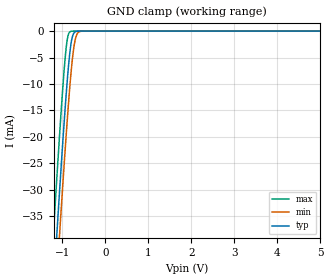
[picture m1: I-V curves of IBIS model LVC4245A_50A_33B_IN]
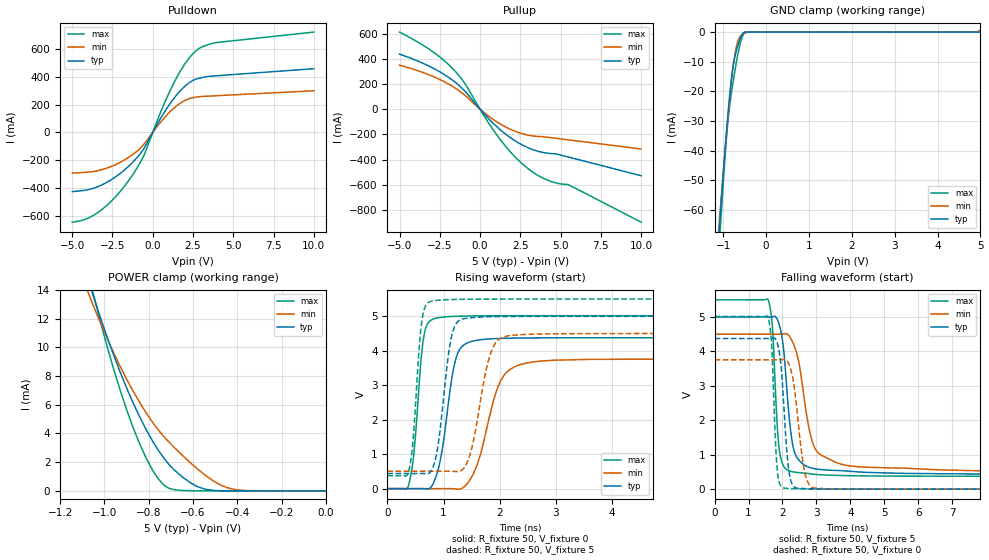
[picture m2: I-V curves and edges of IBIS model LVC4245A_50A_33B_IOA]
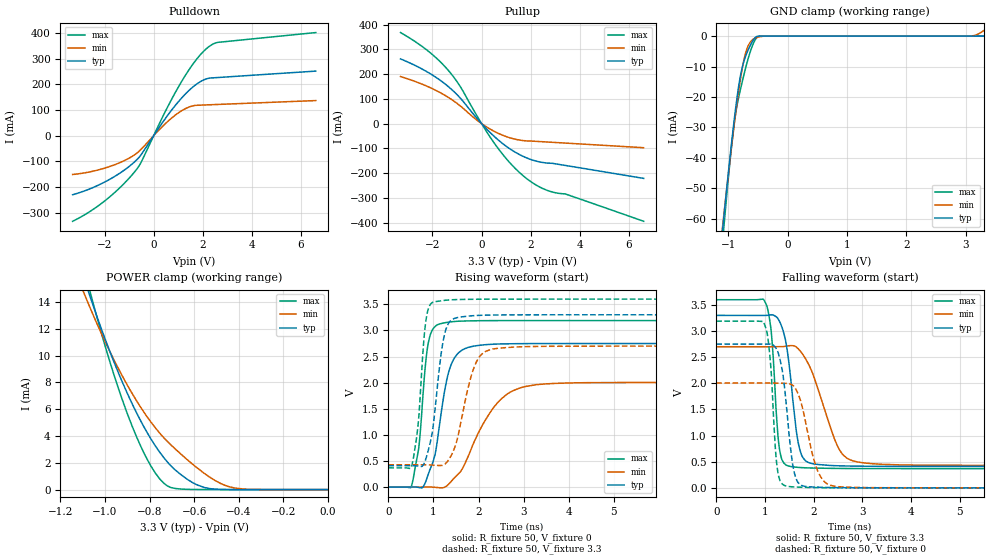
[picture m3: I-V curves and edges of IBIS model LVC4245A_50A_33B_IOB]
| TEXAS INSTRUMENTS INCORPORATED
| Standard Linear and Logic Group
| IBIS Model of SN74LVC4245A
| Octal Bus Transceiver And 3.3-V to 5-V Shifter With 3 state Outputs
| This file contains package information for the following:
|  SSOP 24-pin (DB) package as [Component] LVC4245A_DB
|  SOIC 24-pin (DW) package as [Component] LVC4245A_DW
|  TSSOP 24-pin (PW) package as [Component] LVC4245A_PW
| This device can be powered at the A side at the following Vcca:
|  5 volt Vcca
| This device can be powered at the B side at the following Vccb:
|  3.3 volt Vccb
| This file provides unique models under the [Model Selector] for each Vcc.
| For operation at a specific Vcc, select the appropriate model after each
| [Model Selector] keyword.
[IBIS Ver]   3.2
[Comment char]  |_char
[File Name]   sn74lvc4245a.ibs
[File Rev]   1.0 | b_die
[Date]   March 09, 2001
[Source]   Data created from TI-SPICE simulations at TI-SLL.
[Notes]   The following is an IBIS list for the LVC4245A.
   Please contact sllibis@ti.com with questions and
   comments concerning SLL IBIS models.
   - This device is a 3.3V to 5.0V level shifter, so
   we used the Model selector key word to distinguish
   each model with VCCA and VCCB.
[Disclaimer] Property of Texas Instruments Incorporated.  Unauthorized
   reproduction and/or distribution is strictly prohibited.
   This product is protected under copyright law.
   Created  2001, (C) Copyright  2001, Texas Instruments
   Incorporated, All Rights Reserved
   UNLESS THERE IS A SIGNED, WRITTEN AGREEMENT TO THE
   CONTRARY, TEXAS INSTRUMENTS (TI) IS PROVIDING THE IBIS
   MODELS  AND WITHOUT ANY WARRANTY, EXPRESSED OR
   IMPLIED.  TI assumes no liability for:
   1) the accuracy of the IBIS models provided to your
   company;
   2) the proper functioning of these IBIS Models in your
   design or for any resulting applications; or
   3) infringement of patents, copyrights or intellectual
   property rights resulting from your use of these IBIS
   models.
   TI provides IBIS Models as a service to our customers.
   You and your company shall not distribute, sell or give
   these models to anyone else without prior written
   permission from TI.
   TI reserves the right to make changes to our products or
   to discontinue any semiconductor product or service
   without notice, and advises our customers to obtain the
   latest version of relevant information to verify, before
   placing orders, that the information being relied on is
   current.
   Please be aware that your receipt and use of the IBIS
   information provided shall serve as acceptance of these
   terms and conditions.  If you do not accept these terms,
   you should return or destroy the IBIS models and any
   other accompanying information immediately.
| Component LVC4245A_DB 24-pin SSOP
[Component]   LVC4245A_DB
[Manufacturer]   Texas Instruments, Inc.
[Package]
|   typ   min   max
R_pkg   4.500e-02   4.000e-02   4.900e-02
L_pkg   3.668e-09   3.226e-09   4.415e-09
C_pkg   4.160e-13   3.490e-13   5.070e-13
[Pin]   signal_name   model_name   R_pin   L_pin   C_pin
1   VCCA   POWER   4.200e-02   4.299e-09   5.030e-13
2   DIR   LVC4245A_IN   4.000e-02   3.960e-09   4.990e-13
3   A1   LVC4245A_IOA   4.200e-02   3.775e-09   4.170e-13
4   A2   LVC4245A_IOA   4.700e-02   3.487e-09   3.690e-13
5   A3   LVC4245A_IOA   4.600e-02   3.347e-09   3.520e-13
6   A4   LVC4245A_IOA   4.900e-02   3.352e-09   3.710e-13
7   A5   LVC4245A_IOA   4.600e-02   3.226e-09   3.630e-13
8   A6   LVC4245A_IOA   4.700e-02   3.289e-09   3.490e-13
9   A7   LVC4245A_IOA   4.700e-02   3.347e-09   3.610e-13
10   A8   LVC4245A_IOA   4.100e-02   3.576e-09   4.090e-13
11   GND   GND   4.100e-02   3.995e-09   5.030e-13
12   GND   GND   4.500e-02   4.415e-09   5.070e-13
13   GND   GND   4.300e-02   4.337e-09   5.060e-13
14   B8   LVC4245A_IOB   4.200e-02   4.003e-09   5.040e-13
15   B7   LVC4245A_IOB   4.100e-02   3.686e-09   4.100e-13
16   B6   LVC4245A_IOB   4.800e-02   3.355e-09   3.490e-13
17   B5   LVC4245A_IOB   4.700e-02   3.301e-09   3.530e-13
18   B4   LVC4245A_IOB   4.800e-02   3.268e-09   3.660e-13
19   B3   LVC4245A_IOB   4.800e-02   3.269e-09   3.660e-13
20   B2   LVC4245A_IOB   4.700e-02   3.314e-09   3.490e-13
21   B1   LVC4245A_IOB   4.800e-02   3.399e-09   3.550e-13
22   OE   LVC4245A_IN   4.100e-02   3.688e-09   4.120e-13
23   VCCB   POWER   4.200e-02   4.003e-09   5.040e-13
24   VCCB   POWER   4.300e-02   4.347e-09   5.050e-13
| Component LVC4245A_DW 24-pin SOIC
[Component]   LVC4245A_DW
[Manufacturer]   Texas Instruments, Inc.
[Package]
|   typ   min   max
R_pkg   3.700e-02   3.000e-02   4.700e-02
L_pkg   5.146e-09   3.993e-09   6.885e-09
C_pkg   7.580e-13   5.120e-13   1.067e-12
[Pin]   signal_name   model_name   R_pin   L_pin   C_pin
1   VCCA   POWER   3.900e-02   6.885e-09   1.067e-12
2   DIR   LVC4245A_IN   4.200e-02   5.950e-09   9.580e-13
3   A1   LVC4245A_IOA   4.700e-02   5.317e-09   7.910e-13
4   A2   LVC4245A_IOA   3.100e-02   4.651e-09   6.110e-13
5   A3   LVC4245A_IOA   3.000e-02   3.993e-09   5.120e-13
6   A4   LVC4245A_IOA   3.000e-02   4.083e-09   6.110e-13
7   A5   LVC4245A_IOA   3.000e-02   4.083e-09   6.110e-13
8   A6   LVC4245A_IOA   3.000e-02   3.993e-09   5.120e-13
9   A7   LVC4245A_IOA   3.100e-02   4.652e-09   6.110e-13
10   A8   LVC4245A_IOA   4.700e-02   5.317e-09   7.910e-13
11   GND   GND   4.200e-02   5.950e-09   9.590e-13
12   GND   GND   3.900e-02   6.885e-09   1.067e-12
13   GND   GND   3.900e-02   6.885e-09   1.067e-12
14   B8   LVC4245A_IOB   4.200e-02   5.950e-09   9.590e-13
15   B7   LVC4245A_IOB   4.700e-02   5.317e-09   7.910e-13
16   B6   LVC4245A_IOB   3.100e-02   4.652e-09   6.110e-13
17   B5   LVC4245A_IOB   3.000e-02   3.993e-09   5.120e-13
18   B4   LVC4245A_IOB   3.000e-02   4.083e-09   6.100e-13
19   B3   LVC4245A_IOB   3.000e-02   4.083e-09   6.100e-13
20   B2   LVC4245A_IOB   3.000e-02   3.993e-09   5.120e-13
21   B1   LVC4245A_IOB   3.100e-02   4.651e-09   6.110e-13
22   OE   LVC4245A_IN   4.700e-02   5.317e-09   7.910e-13
23   VCCB   POWER   4.200e-02   5.950e-09   9.580e-13
24   VCCB   POWER   3.900e-02   6.885e-09   1.067e-12
| Component LVC4245A_PW 24-pin TSSOP
[Component]   LVC4245A_PW
[Manufacturer]   Texas Instruments, Inc.
[Package]
|   typ   min   max
R_pkg   3.900e-02   3.000e-02   4.600e-02
L_pkg   2.685e-09   2.367e-09   3.177e-09
C_pkg   3.200e-13   2.520e-13   4.340e-13
[Pin]   signal_name   model_name   R_pin   L_pin   C_pin
1   VCCA   POWER   3.700e-02   3.153e-09   4.340e-13
2   DIR   LVC4245A_IN   3.400e-02   2.629e-09   3.410e-13
3   A1   LVC4245A_IOA   3.200e-02   2.860e-09   3.470e-13
4   A2   LVC4245A_IOA   4.200e-02   2.741e-09   2.900e-13
5   A3   LVC4245A_IOA   4.600e-02   2.600e-09   2.620e-13
6   A4   LVC4245A_IOA   4.300e-02   2.414e-09   2.660e-13
7   A5   LVC4245A_IOA   4.200e-02   2.367e-09   2.620e-13
8   A6   LVC4245A_IOA   4.400e-02   2.461e-09   2.520e-13
9   A7   LVC4245A_IOA   4.200e-02   2.543e-09   2.740e-13
10   A8   LVC4245A_IOA   3.000e-02   2.616e-09   3.320e-13
11   GND   GND   3.700e-02   2.670e-09   3.460e-13
12   GND   GND   3.900e-02   3.177e-09   4.330e-13
13   GND   GND   3.700e-02   3.111e-09   4.310e-13
14   B8   LVC4245A_IOB   3.700e-02   2.656e-09   3.450e-13
15   B7   LVC4245A_IOB   3.100e-02   2.739e-09   3.400e-13
16   B6   LVC4245A_IOB   4.200e-02   2.649e-09   2.820e-13
17   B5   LVC4245A_IOB   4.600e-02   2.532e-09   2.570e-13
18   B4   LVC4245A_IOB   4.400e-02   2.425e-09   2.660e-13
19   B3   LVC4245A_IOB   4.400e-02   2.425e-09   2.660e-13
20   B2   LVC4245A_IOB   4.600e-02   2.532e-09   2.570e-13
21   B1   LVC4245A_IOB   4.200e-02   2.648e-09   2.820e-13
22   OE   LVC4245A_IN   3.100e-02   2.738e-09   3.390e-13
23   VCCB   POWER   3.600e-02   2.653e-09   3.440e-13
24   VCCB   POWER   3.700e-02   3.110e-09   4.310e-13
| Model LVC4245A_IN
[Model Selector]   LVC4245A_IN
LVC4245A_50A_33B_IN   5 volt Vcca, 3.3 volt Vccb
| Model LVC4245A_IOA
[Model Selector]   LVC4245A_IOA
LVC4245A_50A_33B_IOA   5 volt Vcca, 3.3 volt Vccb
| Model LVC4245A_IOB
[Model Selector]   LVC4245A_IOB
LVC4245A_50A_33B_IOB   5 volt Vcca, 3.3 volt Vccb
| Models and submodels in the file (3): LVC4245A_50A_33B_IN (Input), LVC4245A_50A_33B_IOA (I/O), LVC4245A_50A_33B_IOB (I/O)
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[Model]   LVC4245A_50A_33B_IN
Model_type  Input
Vinl=0.8
Vinh=2.0
| variable   typ   min   max
C_comp   2.91pF   2.28pF   4.02pF
[Temperature Range]   40   100   -40
| Ambient temperature   25   85   -40
[Voltage range]   5   4.5   5.5
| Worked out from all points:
|   GND clamp passes 1 mA (typ) near -0.77 V on its own axis
[GND Clamp]
| LVC4245A_50A_33B_IN
|   Voltage   I(typ)   I(min)   I(max)
-5V       -583.8mA   -590.8mA   -575.1mA
-1.21V    -48.93mA   -57.22mA   -38.3mA
-1.13V    -38.42mA   -46.71mA   -27.77mA
-1.07V    -30.71mA   -38.96mA   -20.13mA
-1.05V    -28.19mA   -36.42mA   -17.65mA
-915mV    -12.21mA   -19.95mA   -3.333mA
-870mV    -7.651mA   -14.9mA    -891.1uA
-815mV    -3.252mA   -9.299mA   -87.06uA
-770mV    -1.128mA   -5.445mA   -10.73uA
-705mV    -146.7uA   -1.723mA   -505nA
-575mV    -1.597uA   -52.97uA   -1.115nA
5V        11.12pA    13.99pA    10.67pA
[Model]   LVC4245A_50A_33B_IOA
Model_type  I/O
Vinl=0.8
Vinh=2.0
Enable   Active-Low
Vref =   0
Rref =   500
Cref =   50p
Vmeas =   2.5
| variable   typ   min   max
C_comp   6.39pF   5.64pF   7.42pF
| C_pullup   8.65pF   6.25pF   11.09pF
| C_pulldown   9.51pF   6.70pF   12.70pF
| C_tri-state   6.39pF   5.64pF   7.42pF
[Temperature Range]   40   100   -40
| Ambient temperature   25   85   -40
[Voltage range]   5   4.5   5.5
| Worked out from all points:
|   slope of the pulldown table from 0 to 0.75 V, typ, clamps not added: 4.99 ohm
|   slope of the pullup table from 0 to 0.75 V, typ, clamps not added: 7.23 ohm
|   GND clamp passes 1 mA (typ) near -0.57 V on its own axis
|   POWER clamp passes 1 mA (typ) near -0.65 V on its own axis
|   rising waveform, R_fixture 50, V_fixture 0: 20-80 % time 233ps typ, 372ps min, 145ps max; typ from 0 V to 4.38 V
|   falling waveform, R_fixture 50, V_fixture 5: 20-80 % time 260ps typ, 428ps min, 161ps max; typ from 5 V to 0.439 V
|   rising waveform, R_fixture 50, V_fixture 5: 20-80 % time 195ps typ, 276ps min, 130ps max; typ from 0.439 V to 5 V
|   falling waveform, R_fixture 50, V_fixture 0: 20-80 % time 183ps typ, 268ps min, 124ps max; typ from 4.38 V to 0 V
[GND Clamp]
| LVC4245A_50A_33B_IOA
|   Voltage   I(typ)   I(min)   I(max)
-5V       -990.8mA   -904mA     -1.133A
-1.105V   -68.76mA   -66.5mA    -74.75mA
-1.075V   -62.63mA   -60.92mA   -67.75mA
-1.045V   -56.59mA   -55.42mA   -60.87mA
-965mV    -41.02mA   -41.2mA    -43.47mA
-905mV    -30.14mA   -31.09mA   -32.22mA
-795mV    -14mA      -14.76mA   -19.16mA
-740mV    -9.123mA   -8.534mA   -14.14mA
-680mV    -5.553mA   -4.089mA   -9.05mA
-595mV    -1.866mA   -1.262mA   -3.378mA
-515mV    -93.33uA   -471.4uA   -382.7uA
5V        45pA       618.1uA    384.8pA
[POWER Clamp]
| LVC4245A_50A_33B_IOA
|   Voltage   I(typ)   I(min)   I(max)
-5V       454.4mA    376.9mA    595.8mA
-1.08V    15.04mA    14.07mA    15.61mA
-1.055V   13.81mA    13.09mA    14.01mA
-1.03V    12.62mA    12.14mA    12.49mA
-930mV    8.315mA    8.705mA    7.063mA
-870mV    6.111mA    6.934mA    4.391mA
-810mV    4.22mA     5.398mA    2.229mA
-730mV    2.25mA     3.754mA    387.5uA
-645mV    933.3uA    2.433mA    26.61uA
-580mV    299.7uA    1.53mA     6.704uA
-445mV    3.728uA    222.3uA    613.6nA
-84.45fV  45pA       271.2pA    698.4pA
[Pulldown]
| LVC4245A_50A_33B_IOA
|   Voltage   I(typ)   I(min)   I(max)
-5V       -426.2mA   -292.8mA   -646.2mA
-4.135V   -415.2mA   -287.2mA   -622.9mA
-3.3V     -385.3mA   -272.7mA   -567.6mA
-2.4V     -327.3mA   -236.6mA   -474.2mA
-1.51V    -245.1mA   -180.9mA   -349.2mA
-585mV    -123.1mA   -90.56mA   -174.8mA
575mV     117.8mA    85.67mA    169.1mA
1.395V    256.5mA    182.2mA    374.4mA
2.095V    341.6mA    235mA      509.2mA
2.745V    385.3mA    254.3mA    592.3mA
3.965V    407.1mA    263.6mA    646mA
10V       457.9mA    299.1mA    721.3mA
[Pullup]
| LVC4245A_50A_33B_IOA
|   Voltage   I(typ)   I(min)   I(max)
-5V       437.2mA    349.4mA    612.2mA
-3.03V    333mA      265.5mA    464.7mA
-2.265V   278.5mA    220.6mA    390.1mA
-1.62V    221.3mA    173.6mA    312.1mA
-910mV    138.8mA    106.9mA    197.6mA
330mV     -47.86mA   -35.33mA   -69.57mA
1.175V    -154.6mA   -111.6mA   -228.1mA
2.065V    -242.4mA   -169.8mA   -364.6mA
2.955V    -304.9mA   -205.4mA   -469.8mA
4.21V     -350.2mA   -223.6mA   -565.2mA
5.47V     -380mA     -243.7mA   -599mA
10V       -529mA     -316.4mA   -897.9mA
[Ramp]
| LVC4245A_50A_33B_IOA
| variable   typ   min   max
dV/dt_r   2.63/2.37E-10   2.26/3.79E-10   3.02/1.47E-10
dV/dt_f   2.75/2.64E-10   2.41/4.32E-10   3.09/1.65E-10
R_load = 50
[Rising Waveform]
| LVC4245A_50A_33B_IOA
R_fixture =   50
C_fixture =   0
L_fixture =   0
V_fixture =   0
V_fixture_min = 0
V_fixture_max = 0
|   Time   V(typ)   V(min)   V(max)
0s        -55.47nV   110nV      -22.98nV
385ps     -24.65uV   -72.6nV    147.7mV
475ps     -71.49uV   -773.7nV   1.089V
635ps     -45.98uV   3.583uV    4.278V
790ps     74.24mV    -57.25uV   4.901V
1.09ns    2.55V      1.08mV     4.99V
1.39ns    4.202V     88.04mV    5.008V
2.075ns   4.362V     3.287V     5.016V
2.975ns   4.376V     3.727V     5.017V
49.99ns   4.376V     3.757V     5.017V
[Falling Waveform]
| LVC4245A_50A_33B_IOA
R_fixture =   50
C_fixture =   0
L_fixture =   0
V_fixture =   5
V_fixture_min = 4.5
V_fixture_max = 5.5
|   Time   V(typ)   V(min)   V(max)
0s        5V         4.5V       5.5V
1.57ns    4.999V     4.5V       5.508V
1.695ns   5.005V     4.499V     4.792V
1.855ns   4.912V     4.498V     1.701V
1.955ns   4.577V     4.502V     881.5mV
2.325ns   1.18V      4.213V     500.4mV
2.91ns    601.8mV    1.298V     434.3mV
3.92ns    525.9mV    685.2mV    392.5mV
7.635ns   443.1mV    536.7mV    376.2mV
49.99ns   438.6mV    504.4mV    376.1mV
[Rising Waveform]
| LVC4245A_50A_33B_IOA
R_fixture =   50
C_fixture =   0
L_fixture =   0
V_fixture =   5
V_fixture_min = 4.5
V_fixture_max = 5.5
|   Time   V(typ)   V(min)   V(max)
0s        438.6mV    504.4mV    376.1mV
370ps     438.6mV    504.4mV    455.4mV
630ps     438.7mV    504.4mV    5.034V
830ps     711.6mV    504.4mV    5.453V
970ps     2.174V     504.6mV    5.474V
1.24ns    4.825V     495.1mV    5.49V
1.475ns   4.957V     1.013V     5.495V
1.885ns   4.989V     4.116V     5.499V
2.405ns   4.998V     4.469V     5.5V
49.99ns   5V         4.5V       5.5V
[Falling Waveform]
| LVC4245A_50A_33B_IOA
R_fixture =   50
C_fixture =   0
L_fixture =   0
V_fixture =   0
V_fixture_min = 0
V_fixture_max = 0
|   Time   V(typ)   V(min)   V(max)
0s        4.376V     3.757V     5.017V
1.57ns    4.376V     3.757V     5.006V
1.68ns    4.38V      3.757V     4.172V
1.855ns   4.211V     3.758V     471.6mV
1.965ns   3.507V     3.762V     77.4mV
2.095ns   1.552V     3.752V     26.24mV
2.3ns     113.2mV    3.248V     15.46mV
2.655ns   16.88mV    504mV      4.361mV
3ns       8.527mV    25.7mV     1.608mV
49.99ns   79.05nV    263.1nV    64.55nV
[Model]   LVC4245A_50A_33B_IOB
Model_type  I/O
Vinl=0.8
Vinh=2.0
Enable   Active-Low
Vref =   0
Rref =   500
Cref =   50p
Vmeas =   1.5
| variable   typ   min   max
C_comp   6.96pF   6.03pF   7.82pF
| C_pullup   9.48pF   6.05pF   12.02pF
| C_pulldown   8.35pF   6.84pF   10.36pF
| C_tri-state   6.96pF   6.03pF   7.82pF
[Temperature Range]   40   100   -40
| Ambient temperature   25   85   -40
[Voltage range]   3.3   2.7   3.6
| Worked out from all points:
|   slope of the pulldown table from 0 to 0.495 V, typ, clamps not added: 7.14 ohm
|   slope of the pullup table from 0 to 0.495 V, typ, clamps not added: 9.9 ohm
|   GND clamp passes 1 mA (typ) near -0.57 V on its own axis
|   POWER clamp passes 1 mA (typ) near -0.65 V on its own axis
|   rising waveform, R_fixture 50, V_fixture 0: 20-80 % time 325ps typ, 739ps min, 197ps max; typ from 0 V to 2.75 V
|   falling waveform, R_fixture 50, V_fixture 3.3: 20-80 % time 218ps typ, 496ps min, 133ps max; typ from 3.3 V to 0.409 V
|   rising waveform, R_fixture 50, V_fixture 3.3: 20-80 % time 239ps typ, 364ps min, 165ps max; typ from 0.409 V to 3.3 V
|   falling waveform, R_fixture 50, V_fixture 0: 20-80 % time 189ps typ, 302ps min, 126ps max; typ from 2.75 V to 0 V
[GND Clamp]
| LVC4245A_50A_33B_IOB
|   Voltage   I(typ)   I(min)   I(max)
-3.3V     -549.3mA   -507.9mA   -618.4mA
-1.1V     -64.75mA   -63.66mA   -68.83mA
-1.075V   -59.86mA   -59.17mA   -63.31mA
-1.055V   -55.98mA   -55.61mA   -58.95mA
-910mV    -29.51mA   -31.04mA   -30.47mA
-860mV    -21.56mA   -23.33mA   -23.76mA
-800mV    -13.75mA   -15mA      -18.1mA
-735mV    -8.302mA   -7.85mA    -12.71mA
-675mV    -5.069mA   -3.743mA   -8.169mA
-515mV    -105.9uA   -467.3uA   -422.2uA
3.055V    24.87pA    19.28uA    304.2pA
3.3V      27.13pA    1.796mA    329.3pA
[POWER Clamp]
| LVC4245A_50A_33B_IOB
|   Voltage   I(typ)   I(min)   I(max)
-3.3V     226.7mA    185.8mA    298.2mA
-1.1V     16.06mA    14.88mA    16.91mA
-1.065V   14.3mA     13.48mA    14.63mA
-960mV    9.528mA    9.678mA    8.565mA
-875mV    6.286mA    7.077mA    4.596mA
-795mV    3.804mA    5.057mA    1.782mA
-735mV    2.355mA    3.844mA    458.5uA
-685mV    1.463mA    3.033mA    83.96uA
-590mV    373.6uA    1.662mA    8.133uA
-505mV    32.25uA    665.2uA    1.757uA
-440mV    3.104uA    198.4uA    564.7nA
-48.03fV  27.13pA    253pA      621.9pA
[Pulldown]
| LVC4245A_50A_33B_IOB
|   Voltage   I(typ)   I(min)   I(max)
-3.3V     -229.6mA   -150.8mA   -332.9mA
-2.6V     -206.8mA   -140.7mA   -295.1mA
-1.905V   -175.6mA   -123.4mA   -247mA
-1.28V    -139.4mA   -100.7mA   -193.3mA
-705mV    -95.23mA   -69.29mA   -132.3mA
-500mV    -72.46mA   -51.72mA   -101.5mA
410mV     57.97mA    40.88mA    81.79mA
1.03V     134.8mA    90.37mA    193.2mA
1.67V     195.1mA    117.5mA    287.7mA
2.225V    223.1mA    120.1mA    344.6mA
2.635V    226.4mA    121.7mA    363.4mA
6.6V      251.3mA    136.7mA    401.2mA
[Pullup]
| LVC4245A_50A_33B_IOB
|   Voltage   I(typ)   I(min)   I(max)
-3.3V     261.4mA    190.1mA    367.8mA
-2.205V   208.4mA    150.2mA    295.4mA
-1.37V    150.9mA    106.8mA    216.8mA
-875mV    103.9mA    72.02mA    150.7mA
-90mV     10.07mA    6.442mA    14.99mA
585mV     -58.1mA    -34.86mA   -88.41mA
1.21V     -105.8mA   -59.11mA   -164.7mA
1.835V    -138.7mA   -69.94mA   -222.2mA
2.26V     -152.5mA   -72.04mA   -250.6mA
2.685V    -159.6mA   -74.52mA   -270.3mA
3.4V      -169mA     -78.71mA   -284.1mA
6.6V      -221.5mA   -97.53mA   -394.9mA
[Ramp]
| LVC4245A_50A_33B_IOB
| variable   typ   min   max
dV/dt_r   1.66/3.33E-10   1.21/7.60E-10   1.92/2.00E-10
dV/dt_f   1.74/2.27E-10   1.38/5.03E-10   1.95/1.36E-10
R_load = 50
[Rising Waveform]
| LVC4245A_50A_33B_IOB
R_fixture =   50
C_fixture =   0
L_fixture =   0
V_fixture =   0
V_fixture_min = 0
V_fixture_max = 0
|   Time   V(typ)   V(min)   V(max)
0s        -2.059uV   -7.324uV   -460.2nV
515ps     856.3uV    -23.01uV   28.17mV
675ps     -7.337mV   193.1uV    759.6mV
795ps     39.75mV    1.465mV    2.074V
980ps     460.1mV    -463.8uV   3.016V
1.295ns   2.055V     23.11mV    3.154V
1.495ns   2.51V      203.1mV    3.174V
2.5ns     2.742V     1.686V     3.189V
3.705ns   2.749V     1.986V     3.189V
50ns      2.75V      2.005V     3.189V
[Falling Waveform]
| LVC4245A_50A_33B_IOB
R_fixture =   50
C_fixture =   0
L_fixture =   0
V_fixture =   3.3
V_fixture_min = 2.7
V_fixture_max = 3.6
|   Time   V(typ)   V(min)   V(max)
0s        3.3V       2.7V       3.6V
1.005ns   3.3V       2.7V       3.55V
1.125ns   3.31V      2.7V       3.018V
1.25ns    3.258V     2.701V     1.192V
1.31ns    3.161V     2.702V     676.6mV
1.45ns    2.669V     2.712V     429mV
1.71ns    750.1mV    2.633V     389.7mV
2.565ns   420.7mV    675.4mV    371mV
3.41ns    411.8mV    450.5mV    368.6mV
50ns      409mV      427mV      368.3mV
[Rising Waveform]
| LVC4245A_50A_33B_IOB
R_fixture =   50
C_fixture =   0
L_fixture =   0
V_fixture =   3.3
V_fixture_min = 2.7
V_fixture_max = 3.6
|   Time   V(typ)   V(min)   V(max)
0s        409mV      427mV      368.3mV
525ps     409.3mV    427.1mV    429.6mV
670ps     400.4mV    427.2mV    1.295V
805ps     477.1mV    427.4mV    2.989V
935ps     879.3mV    424.2mV    3.506V
1.195ns   2.699V     415.5mV    3.571V
1.345ns   3.152V     533.3mV    3.584V
1.985ns   3.288V     2.452V     3.598V
2.81ns    3.299V     2.683V     3.6V
50ns      3.3V       2.7V       3.6V
[Falling Waveform]
| LVC4245A_50A_33B_IOB
R_fixture =   50
C_fixture =   0
L_fixture =   0
V_fixture =   0
V_fixture_min = 0
V_fixture_max = 0
|   Time   V(typ)   V(min)   V(max)
0s        2.75V      2.005V     3.189V
975ps     2.751V     2.006V     3.163V
1.1ns     2.752V     2.006V     2.522V
1.21ns    2.692V     2.004V     792.5mV
1.265ns   2.599V     2.003V     293mV
1.375ns   2.122V     2.001V     58.8mV
1.575ns   409.8mV    1.957V     18.56mV
2.105ns   12.3mV     276.3mV    4.916mV
2.61ns    3.885mV    15.33mV    979uV
50ns      -1.858uV   -7.332uV   -324.6nV
